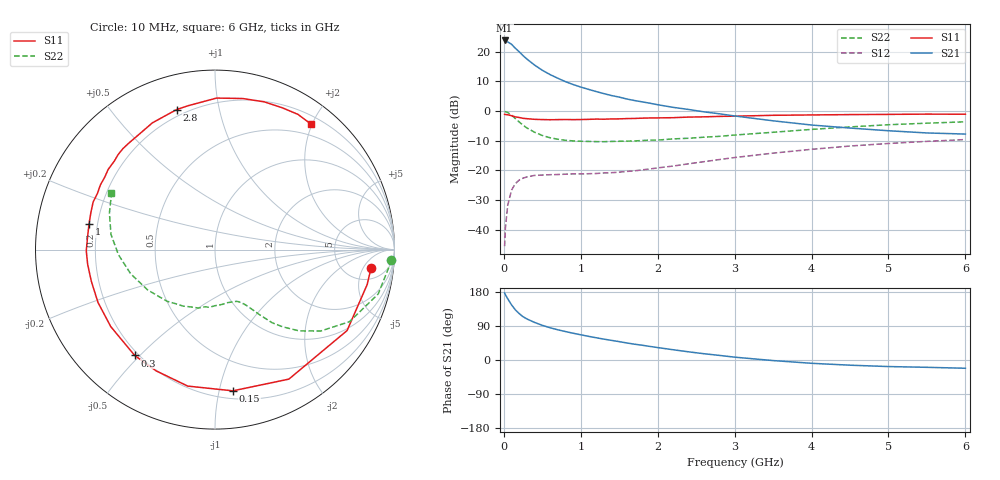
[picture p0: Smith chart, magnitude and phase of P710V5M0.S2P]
! SIEMENS Small Signal Semiconductors
! BFP196
! Si NPN RF Bipolar Junction Transistor in SOT143
! VCE = 10 V  IC = 5 mA
! Common Emitter S-Parameters:  May  1996
# GHz  S  MA  R  50
!  f  S11  S21  S12  S22
! GHz  MAG  ANG  MAG  ANG  MAG  ANG  MAG  ANG
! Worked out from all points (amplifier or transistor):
!   36 points, 10 MHz to 6 GHz, reference 50 ohm
!   highest |S21| = 23.7 dB at 10 MHz (marker M1)
!   |S21| within 3 dB of that: start of sweep to 165.5 MHz
!   unconditionally stable (mu >= 1): 1.19 GHz to 3.256 GHz
!   at 250 MHz: K = 0.25, MSG = 20.6 dB, |S12| = -22.6 dB
!   at 1.4 GHz: K = 1.13, MAG = 10.8 dB, |S12| = -20.8 dB
!   at 6 GHz: K = 0.98, MSG = 0.9 dB, |S12| = -9.6 dB
!   S11 on the Smith chart (normalised r, x): 10 MHz: 9, -7; 150 MHz: 0.26, -1.10; 300 MHz: 0.18, -0.48; 1 GHz: 0.17, +0.10; 2.8 GHz: 0.17, +0.75; 6 GHz: 0.32, +1.97
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0.01  0.8757 -6.6  15.34 177.1  0.0053 86.0  0.982 -3.3
0.02  0.87 -12.9  14.94 172.3  0.0106 82.3  0.9718 -6.2
0.05  0.8631 -31.5  14.52 161.7  0.0257 73.2  0.9425 -15.2
0.1  0.8308 -60.3  13.23 145.6  0.0465 59.5  0.8502 -28.2
0.15  0.7931 -82.8  11.33 132.2  0.0599 48.4  0.7434 -37.6
0.2  0.7755 -101.3  9.889 122.4  0.0688 41.1  0.6521 -44.0
0.25  0.751 -115.9  8.52 114.2  0.074 35.2  0.573 -48.7
0.3  0.7403 -127.2  7.454 108.3  0.0776 31.7  0.5174 -52.0
0.4  0.7221 -143.6  5.907 99.1  0.0822 26.4  0.4379 -55.7
0.5  0.7153 -155.7  4.835 91.5  0.0834 23.5  0.3864 -58.5
0.6  0.7113 -165.6  4.095 85.2  0.0845 22.3  0.3536 -60.9
0.7  0.7143 -173.4  3.555 79.8  0.0851 21.5  0.3344 -63.1
0.8  0.7172 -179.5  3.114 75.1  0.0862 21.5  0.3205 -65.3
1  0.7161 168.6  2.521 66.5  0.0871 22.6  0.3087 -69.6
1.1  0.7214 163.6  2.308 62.5  0.0878 23.7  0.3067 -72.4
1.6  0.7442 143.1  1.585 44.9  0.096 31.0  0.3103 -87.1
2.2  0.7701 122.8  1.149 27.1  0.1181 37.8  0.3383 -105.7
2.8  0.809 105.3  0.896 12.2  0.1519 39.1  0.3736 -126.4
3.5  0.8443 89.4  0.682 -1.5  0.1949 34.6  0.4374 -149.1
4.5  0.8676 71.6  0.515 -13.7  0.2566 24.0  0.5384 -176.9
5.5  0.8838 58.5  0.426 -19.3  0.3075 11.6  0.6225 160.9
6  0.8804 52.8  0.408 -21.8  0.3297 5.0  0.6562 151.5
